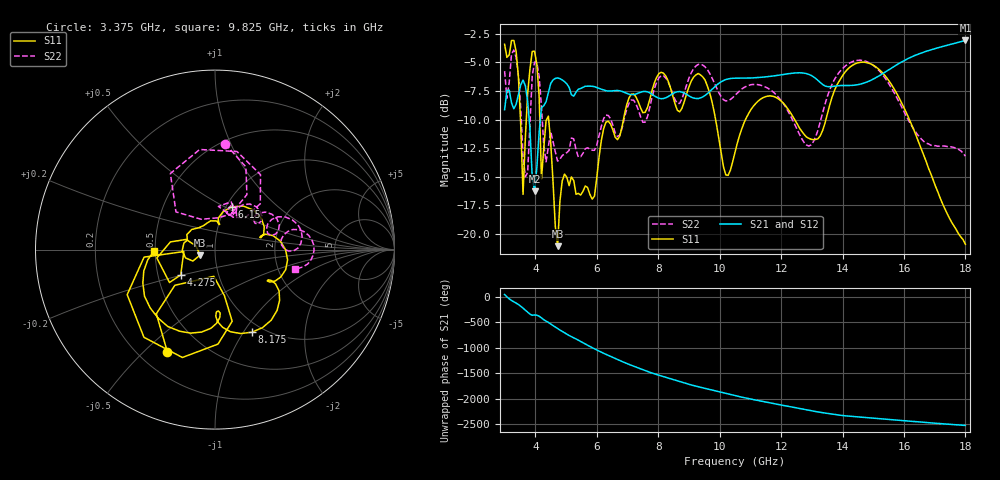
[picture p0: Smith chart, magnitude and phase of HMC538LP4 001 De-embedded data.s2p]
! Chelmsford, MA 01824
! http://www.hittite.com
! Tel: 978-250-3343
! Fax: 978-250-3373
! Device  :  HMC538LP4
! Description:  600 Analog Phase Shifter
! Frequency  :  6.0 GHz - 15.0 GHz
! Package  :  LP4  - 4x4 mm Quad Flatpack No-Lead (QFN) Plastic Package: 24 pin
! Ports  :  2 RF, 1 DC
!  Pin  3  = Rfin  = Port 1
!  Pin  16  = Rfout = Port 2
!  pin  21  = vCTL
! Voltages:  VCTL  = 0 to 5.0 Volts
! Currents :  Vb(V)  Vd(V)  Ib(mA)  Id(mA)
!  0.00  0.10  0.000000  0.483525
! Data:  The device was measured on evaluation board 111296-1.
!  Data was collected using a calibrated network analyzer.
!  The evaluation circuit board was modeled and simulated.This was use
!  to removed the evaluation board circuit from the measured data.
!  The reference plane is the center of the package pin.
! Misc:  Lot #
!Date Measured:  03 - 11 -2009
! Date:  03 - 17 -2009
! Note:
!  Hittite Microwave supplies this data as a sample of measured data at the
!  package pin for this package product.  Your particular data for this product
!  may vary.
!  Data was taken at 25 degrees C.
!  Hittite Microwave reserves the right to change this data at anytime.
# MHz S MA R 50
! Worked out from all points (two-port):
!   201 points, 3 GHz to 18 GHz, reference 50 ohm
!   highest |S21| = -3.09 dB at 18 GHz (marker M1); lowest = -16.3 dB at 3.975 GHz (marker M2)
!   |S21| within 3 dB of the highest: 12 GHz to 12.93 GHz (929.7 MHz wide, 7.46 % of centre); 15.25 GHz to end of sweep
!   lowest |S11| = -21.1 dB at 4.725 GHz (marker M3), VSWR 1.19, Z = 42.3 - j2.62 ohm
!   |S11| at or under -10 dB: 4.435 GHz to 6.868 GHz (2.433 GHz wide, 43.1 % of centre); 12.44 GHz to 13.46 GHz (1.019 GHz wide, 7.87 % of centre); 16.18 GHz to end of sweep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
!   |S22| runs from -15.0 to -3.9 dB; largest |S21 - S12| = 0.002
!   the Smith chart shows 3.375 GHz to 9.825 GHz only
!   S11 on the Smith chart (normalised r, x): 3.375 GHz: 0.31, -0.59; 4.275 GHz: 0.66, -0.20; 6.15 GHz: 1.07, +0.54; 8.175 GHz: 0.89, -1.09; 9.825 GHz: 0.49, -0.01
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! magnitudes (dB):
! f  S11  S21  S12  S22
! 3 GHz  -3.4  -9.1  -9.1  -5.8
! 3.375 GHz  -4.0  -8.7  -8.7  -4.6
! 3.6 GHz  -16.5  -6.5  -6.6  -13.2
! 3.75 GHz  -7.7  -8.4  -8.4  -14.6
! 3.975 GHz  -4.0  -16.3  -16.3  -5.0
! 4.2 GHz  -15.2  -9.0  -9.0  -8.9
! 4.275 GHz  -12.5  -8.8  -8.8  -12.3
! 4.425 GHz  -9.7  -7.6  -7.7  -12.4
! 4.725 GHz  -21.1  -6.4  -6.4  -13.6
! 4.95 GHz  -14.8  -6.7  -6.7  -13.0
! 5.55 GHz  -16.3  -7.2  -7.2  -12.9
! 6.15 GHz  -11.8  -7.3  -7.4  -10.6
! 8.025 GHz  -6.0  -8.1  -8.1  -6.3
! 8.175 GHz  -6.0  -8.2  -8.2  -6.2
! 9.825 GHz  -9.4  -7.2  -7.2  -6.8
! 10.2 GHz  -14.8  -6.5  -6.5  -8.4
! 10.5 GHz  -12.9  -6.4  -6.4  -7.9
! 11.55 GHz  -8.0  -6.3  -6.3  -7.2
! 13.05 GHz  -11.8  -6.3  -6.3  -11.9
! 14.1 GHz  -5.8  -7.0  -7.0  -5.3
! 15.53 GHz  -6.7  -5.6  -5.6  -6.9
! 18 GHz  -20.9  -3.1  -3.1  -13.2
